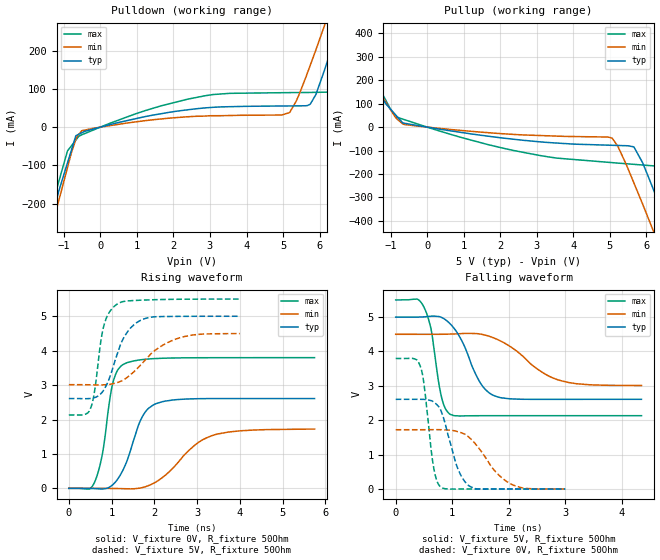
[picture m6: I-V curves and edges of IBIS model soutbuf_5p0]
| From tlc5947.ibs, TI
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|   soutbuf_5p0 Model
[Model]   soutbuf_5p0
Model_type   Output
Polarity   Non-Inverting
Vmeas = 2.5
Vref = 2.5
Cref = 15pF
Rref = 50
|   typ   min   max
|   (nom PVT)   (Fast PVT)   (slow PVT)
|Average
C_comp   2.906e-12   2.890e-12   3.254e-12
|ON state : BUFFER OUTPUT TURNED HIGH
|C_comp   2.906e-12   2.890e-12   3.254e-12
|OFF state: BUFFER OUTPUT TURNED LOW
|C_comp   2.387e-12   2.450e-12   2.236e-12
| Where nom  PVT is Nominal Process,  5V,  65C
|   Fast PVT is Strong Process,   5.5V,  -40C
[Voltage Range]   5   4.5   5.5
|Ambient Temperature   25   85   -40
|Junction Temperature
[Temperature Range]   65   125   -40
[Pullup Reference]   5   4.5   5.5
[Pulldown Reference]   0   0   0
[Power Clamp Reference]   5   4.5   5.5
[GND Clamp Reference]   0   0   0
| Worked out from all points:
|   slope of the pulldown table from 0 to 0.75 V, typ, clamps not added: 42.9 ohm
|   slope of the pullup table from 0 to 0.75 V, typ, clamps not added: 40.8 ohm
|   falling waveform, V_fixture 5V, R_fixture 50Ohm: 20-80 % time 400ps typ, 713ps min, 193ps max; typ from 5 V to 2.61 V
|   rising waveform, V_fixture 0V, R_fixture 50Ohm: 20-80 % time 460ps typ, 865ps min, 279ps max; typ from 0 V to 2.61 V
|   rising waveform, V_fixture 5V, R_fixture 50Ohm: 20-80 % time 446ps typ, 808ps min, 243ps max; typ from 2.61 V to 5 V
|   falling waveform, V_fixture 0V, R_fixture 50Ohm: 20-80 % time 276ps typ, 491ps min, 157ps max; typ from 2.61 V to 0 V
[Pulldown]
|   Voltage   I(typ)   I(min)   I(max)
-5V       -1.775A    -1.704A    -1.911A
-1.369V   -258.4mA   -275.3mA   -234.3mA
-896.5mV  -92.21mA   -104.3mA   -61.48mA
-670mV    -22.3mA    -32.21mA   -33.79mA
-508.5mV  -14.62mA   -9.304mA   -19.91mA
2.376V    45.08mA    27.02mA    72.72mA
5.175V    55.34mA    37.89mA    90.12mA
5.745V    59.89mA    161.5mA    90.55mA
6.13V     147.5mA    264mA      91.18mA
6.501V    257.1mA    366mA      127.5mA
6.89V     377.5mA    475.4mA    262.7mA
10V       1.587A     1.468A     1.75A
[Pullup]
|   Voltage   I(typ)   I(min)   I(max)
-5V       1.515A     1.266A     1.964A
-2.354V   476.3mA    435.6mA    563.4mA
-2.196V   426.5mA    389.8mA    499.7mA
-1.018V   79.03mA    77.6mA     80.02mA
-670.5mV  17.98mA    13.52mA    34.29mA
2.376V    -51.78mA   -31.16mA   -100mA
5.058V    -77.42mA   -46.94mA   -151.3mA
5.66V     -85.22mA   -239.3mA   -158.7mA
6.215V    -276.1mA   -452.9mA   -165.4mA
6.6V      -433.7mA   -603.3mA   -270.9mA
6.88V     -550.2mA   -713mA     -396.2mA
10V       -1.865A    -1.952A    -1.846A
[Ramp]
R_load = 50
|   typ   min   max
dV/dt_r   1.56519/4.59602e-10   1.03452/8.66255e-10   2.2783/2.79212e-10
dV/dt_f   1.43458/3.9957e-10   0.892927/7.11281e-10   2.02063/1.93414e-10
[Falling Waveform]
V_fixture = 5V
V_fixture_min = 4.5V
V_fixture_max = 5.5V
R_fixture = 50Ohm
|   Time   V(typ)   V(min)   V(max)
0s        5V         4.5V       5.5V
375ps     5V         4.5V       5.525V
500ps     5.007V     4.5V       5.292V
625ps     5.025V     4.5V       4.662V
825ps     4.98V      4.501V     2.581V
975ps     4.785V     4.507V     2.164V
1.5ns     3.08V      4.506V     2.132V
1.75ns    2.71V      4.385V     2.133V
2.875ns   2.607V     3.174V     2.133V
4.35ns    2.609V     3.011V     2.133V
[Rising Waveform]
V_fixture = 0V
V_fixture_min = 0V
V_fixture_max = 0V
R_fixture = 50Ohm
|   Time   V(typ)   V(min)   V(max)
0s        549.1pV    3.073nV    461.8pV
600ps     -7.088mV   661.3uV    171.8mV
775ps     -20.07mV   -279.1uV   930.5mV
1.025ns   101.6mV    -3.877mV   3.039V
1.275ns   551.4mV    -9.985mV   3.6V
1.7ns     2.033V     16.07mV    3.738V
2.05ns    2.465V     194.6mV    3.772V
2.975ns   2.603V     1.283V     3.794V
3.4ns     2.609V     1.551V     3.796V
5.75ns    2.609V     1.721V     3.797V
[Rising Waveform]
V_fixture = 5V
V_fixture_min = 4.5V
V_fixture_max = 5.5V
R_fixture = 50Ohm
|   Time   V(typ)   V(min)   V(max)
0s        2.609V     3.012V     2.132V
500ps     2.61V      3.008V     2.299V
600ps     2.636V     3.005V     2.804V
750ps     2.752V     3.004V     4.29V
825ps     2.872V     3.008V     4.751V
1.125ns   3.872V     3.07V      5.348V
1.4ns     4.594V     3.256V     5.447V
1.8ns     4.94V      3.743V     5.473V
2.625ns   4.997V     4.385V     5.494V
4ns       5V         4.498V     5.5V
[Falling Waveform]
V_fixture = 0V
V_fixture_min = 0V
V_fixture_max = 0V
R_fixture = 50Ohm
|   Time   V(typ)   V(min)   V(max)
0s        2.609V     1.724V     3.797V
350ps     2.609V     1.724V     3.774V
450ps     2.608V     1.724V     3.504V
500ps     2.607V     1.725V     3.065V
675ps     2.53V      1.726V     597.5mV
800ps     2.283V     1.725V     55.56mV
1.075ns   700.3mV    1.678V     -1.097mV
1.3ns     89.56mV    1.501V     246.3uV
2.025ns   1.076mV    158mV      416.6uV
3ns       126.8uV    669.8uV    379uV
